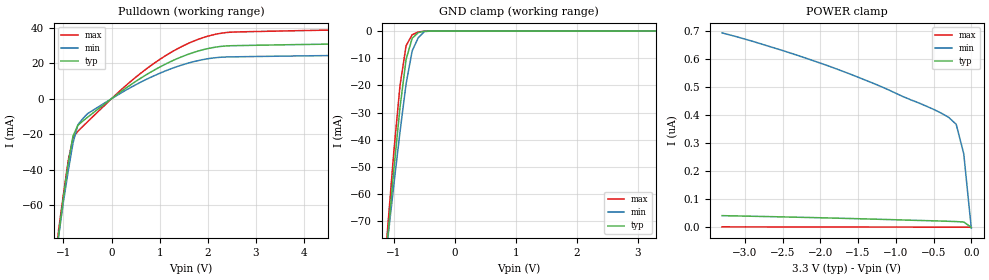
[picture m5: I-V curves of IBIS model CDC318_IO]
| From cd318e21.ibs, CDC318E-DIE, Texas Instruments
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|   Model CDC318_IO
[Model]   CDC318_IO
Model_type   I/O_open_drain
Polarity   Non-Inverting
Vinl = 0.99V
Vinh = 2.31V
Vmeas = 1.5V
Cref = 400pF
Rref = 1000
Vref = 3.3
|   variable   typ   min   max
C_comp   6.2p   NA   NA
[Voltage range]   3.3   3.135   3.465
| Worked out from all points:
|   slope of the pulldown table from 0 to 0.495 V, typ, clamps not added: 51.6 ohm
|   GND clamp passes 1 mA (typ) near -0.62 V on its own axis
[Pulldown]
|  Voltage   I(typ)   I(min)   I(max)
-3.3V     -670.7mA   -564.2mA   -793.1mA
-1.2V     -102mA     -97.14mA   -102.6mA
-1.1V     -77.01mA   -77.49mA   -73.84mA
-900mV    -36.23mA   -40.65mA   -34.81mA
-800mV    -20.96mA   -24.85mA   -21.99mA
-700mV    -15.03mA   -14.73mA   -18.38mA
-500mV    -10.51mA   -8.493mA   -13.05mA
600mV     11.4mA     9.179mA    14.16mA
1.6V      25.04mA    20.06mA    31.16mA
2.1V      28.73mA    22.86mA    35.88mA
2.5V      29.82mA    23.54mA    37.48mA
6.6V      31.47mA    24.87mA    39.52mA
[GND_Clamp]
|  Voltage   I(typ)   I(min)   I(max)
-3.3V     -671.5mA   -564.8mA   -794.1mA
-1.2V     -101.3mA   -96.56mA   -101.7mA
-1.1V     -75.44mA   -76.35mA   -71.74mA
-1V       -50.78mA   -56.32mA   -44.01mA
-900mV    -28.1mA    -37.11mA   -20.01mA
-800mV    -10.41mA   -19.39mA   -5.356mA
-700mV    -2.628mA   -7.244mA   -1.323mA
-600mV    -568.7uA   -2.428mA   -330.9uA
-500mV    -49.49uA   -184.7uA   -37.69uA
3.3V      16.23pA    357.4nA    -425.4nA
[POWER_clamp]
|  Voltage   I(typ)   I(min)   I(max)
-3.3V     41.73nA    693.8nA    1.691nA
-2.5V     37.29nA    631nA      1.46nA
-1.8V     32.88nA    566.8nA    1.242nA
-1.2V     28.61nA    502.9nA    1.046nA
-500mV    23.26nA    421nA      810pA
-300mV    21.61nA    392.6nA    741.9pA
-200mV    20.65nA    367.7nA    703.5pA
-100mV    19.07nA    262.7nA    660.8pA
0V        16.23pA    -2.894nA   408.3pA
[Ramp]
|  variable   typ   min   max
dV/dt_f   1.32/140n   1.25/200n   1.39/90n
dV/dt_r   1.32/1n   1.25/1n   1.39/1n  | internal slope
